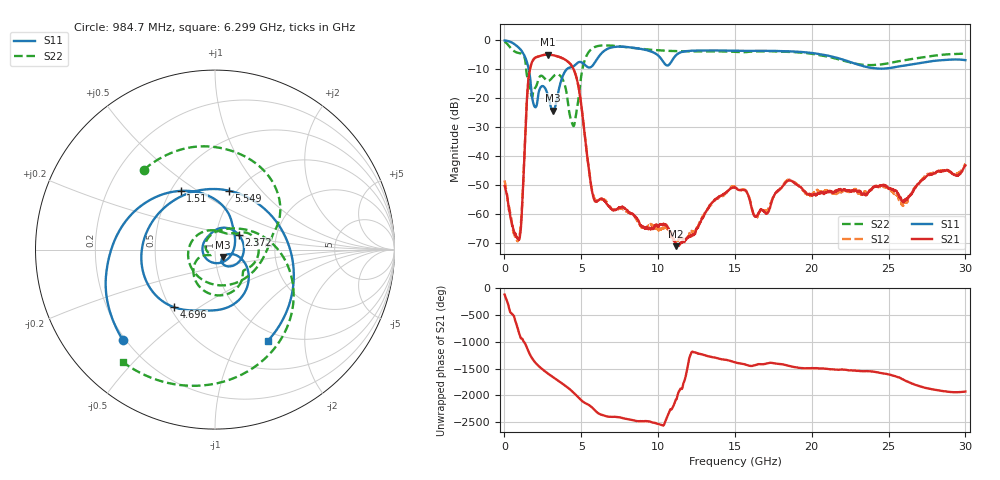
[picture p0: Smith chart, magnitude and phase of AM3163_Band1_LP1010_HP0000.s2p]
!Agilent Technologies,E8364B,MY43040894,A.07.50.67
!Agilent E8364B: A.07.50.67
!Date: Thursday, August 20, 2020 11:30:40
!Correction: S11(Full 2 Port(1,2))
!S21(Full 2 Port(1,2))
!S12(Full 2 Port(1,2))
!S22(Full 2 Port(1,2))
!S2P File: Measurements: S11, S21, S12, S22:
# Hz S  dB  R 50
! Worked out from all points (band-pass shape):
!   3201 points, 10 MHz to 30 GHz, reference 50 ohm
!   highest |S21| = -4.97 dB at 2.803 GHz (marker M1); lowest = -71.2 dB at 11.18 GHz (marker M2)
!   |S21| within 3 dB of the highest: 1.765 GHz to 4.244 GHz (2.479 GHz wide, 82.5 % of centre)
!   lowest |S11| = -24.3 dB at 3.159 GHz (marker M3), VSWR 1.13, Z = 54.5 - j4.53 ohm
!   |S11| at or under -10 dB: 1.58 GHz to 4.062 GHz (2.482 GHz wide, 88 % of centre)
!   |S22| runs from -29.7 to -0.5 dB; largest |S21 - S12| = 0.0063
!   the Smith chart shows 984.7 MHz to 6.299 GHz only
!   S11 on the Smith chart (normalised r, x): 984.7 MHz: 0.19, -0.40; 1.51 GHz: 0.56, +0.43; 2.372 GHz: 1.28, +0.22; 4.696 GHz: 0.53, -0.40; 5.549 GHz: 0.92, +0.68; 6.299 GHz: 0.87, -1.35
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1e7  -0.09 -8.9  -50.36 -118.6  -48.49 16.0  -0.53 -20.6
5.629406e8  -1.06 -75.0  -64.90 -144.2  -65.76 26.4  -3.51 -144.3
9.84675e8  -2.86 -135.6  -68.64 -147.2  -67.42 2.3  -4.49 131.7
1.5095e9  -8.43 120.3  -16.68 -61.3  -16.66 -61.4  -13.48 -67.2
1.949978e9  -22.85 -112.2  -6.29 71.9  -6.29 71.9  -16.84 38.3
2.371712e9  -16.15 32.3  -5.35 -49.3  -5.35 -49.4  -12.28 1.5
2.802819e9  -18.63 -52.8  -4.97 -146.5  -4.97 -146.5  -14.07 -35.6
3.15895e9  -24.30 -42.8  -5.19 140.9  -5.20 140.9  -12.65 -52.0
3.814981e9  -12.14 -40.5  -6.34 10.5  -6.36 10.7  -13.83 -122.4
4.695938e9  -8.11 -125.1  -13.13 155.2  -13.09 155.3  -24.56 154.9
5.014581e9  -7.64 -171.5  -23.04 64.1  -23.00 63.9  -11.74 19.5
5.548778e9  -9.44 76.7  -46.99 -28.7  -46.93 -29.8  -3.65 -62.5
6.298528e9  -4.63 -59.8  -54.75 160.0  -54.94 163.2  -1.83 -129.2
7.751169e9  -2.27 -175.9  -57.85 93.0  -58.48 89.2  -2.30 152.1
1.000979e10  -5.32 72.1  -64.58 -13.8  -65.14 -36.2  -3.49 62.0
1.118128e10  -5.12 63.8  -71.20 84.9  -69.60 67.3  -3.77 20.3
1.5005e10  -3.63 -72.0  -50.91 56.4  -50.71 58.8  -4.02 -93.4
1.636392e10  -3.67 -104.6  -60.91 10.4  -61.46 5.6  -3.86 -124.4
2.000958e10  -4.41 163.3  -53.49 -49.6  -53.15 -52.2  -4.70 136.5
2.275554e10  -8.00 60.3  -52.19 -95.6  -51.51 -99.4  -8.01 21.3
2.500479e10  -9.68 -62.3  -51.41 -169.1  -51.25 -167.3  -7.97 -92.4
3e10  -6.89 104.9  -43.27 -128.0  -42.83 -126.3  -4.66 102.6
